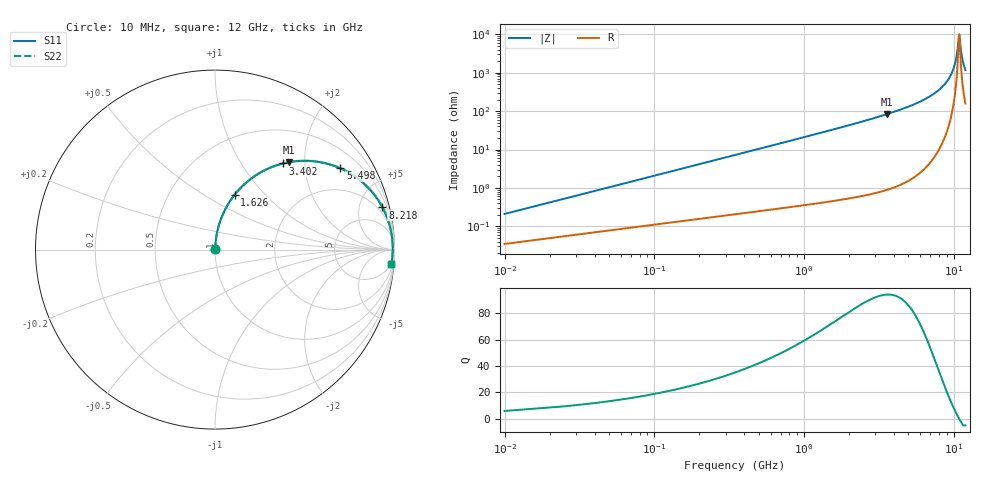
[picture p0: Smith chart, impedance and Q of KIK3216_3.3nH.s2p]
!version-2
!date-01.2022
!Series
# MHz S RI R 50
!Freq ReS11 ImS11 ReS21 ImS21 ReS12 ImS12 ReS22 ImS22
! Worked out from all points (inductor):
!   751 points, 10 MHz to 12 GHz, reference 50 ohm
!   read as one part in series: L = 3.3 nH near 58 MHz
!   highest Q = 94 at 3.594 GHz (marker M1), where L = 3.7 nH
!   self-resonance near 10.91 GHz
!   S11 on the Smith chart (normalised r, x): 10 MHz: 1.00, +0.00; 1.626 GHz: 1.01, +0.69; 3.402 GHz: 1.02, +1.56; 5.498 GHz: 1.04, +3.06; 8.218 GHz: 1.24, +7.87; 12 GHz: 4, -23
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10  0.000352 0.00207  0.9996 -0.00207  0.9996 -0.00207  0.000352 0.00207
74  0.00118 0.0153  0.9988 -0.0153  0.9988 -0.0153  0.00118 0.0153
122  0.00185 0.0252  0.9981 -0.0252  0.9981 -0.0252  0.00185 0.0252
218  0.00365 0.045  0.9963 -0.045  0.9963 -0.045  0.00365 0.045
362  0.00767 0.0744  0.9923 -0.0744  0.9923 -0.0744  0.00767 0.0744
570  0.0164 0.1163  0.9836 -0.1163  0.9836 -0.1163  0.0164 0.1163
842  0.0329 0.1693  0.9671 -0.1693  0.9671 -0.1693  0.0329 0.1693
1626  0.1095 0.3056  0.8905 -0.3056  0.8905 -0.3056  0.1095 0.3056
2010  0.16 0.3605  0.84 -0.3605  0.84 -0.3605  0.16 0.3605
3402  0.3803 0.4802  0.6197 -0.4802  0.6197 -0.4802  0.3803 0.4802
3594  0.4123 0.487  0.5877 -0.487  0.5877 -0.487  0.4123 0.487
4010  0.4805 0.4943  0.5195 -0.4943  0.5195 -0.4943  0.4805 0.4943
5498  0.6979 0.4529  0.3021 -0.4529  0.3021 -0.4529  0.6979 0.4529
6010  0.7588 0.4208  0.2412 -0.4208  0.2412 -0.4208  0.7588 0.4208
8010  0.9223 0.254  0.0777 -0.254  0.0777 -0.254  0.9223 0.254
8218  0.933 0.235  0.067 -0.235  0.067 -0.235  0.933 0.235
9274  0.9717 0.139  0.0283 -0.139  0.0283 -0.139  0.9717 0.139
10010  0.9853 0.0744  0.0147 -0.0744  0.0147 -0.0744  0.9853 0.0744
10490  0.9893 0.034  0.0107 -0.034  0.0107 -0.034  0.9893 0.034
10906  0.99 0.00036  0.00997 -0.00036  0.00997 -0.00036  0.99 0.00036
11386  0.9881 -0.0369  0.0119 0.0369  0.0119 0.0369  0.9881 -0.0369
12000  0.9819 -0.0818  0.0181 0.0818  0.0181 0.0818  0.9819 -0.0818
